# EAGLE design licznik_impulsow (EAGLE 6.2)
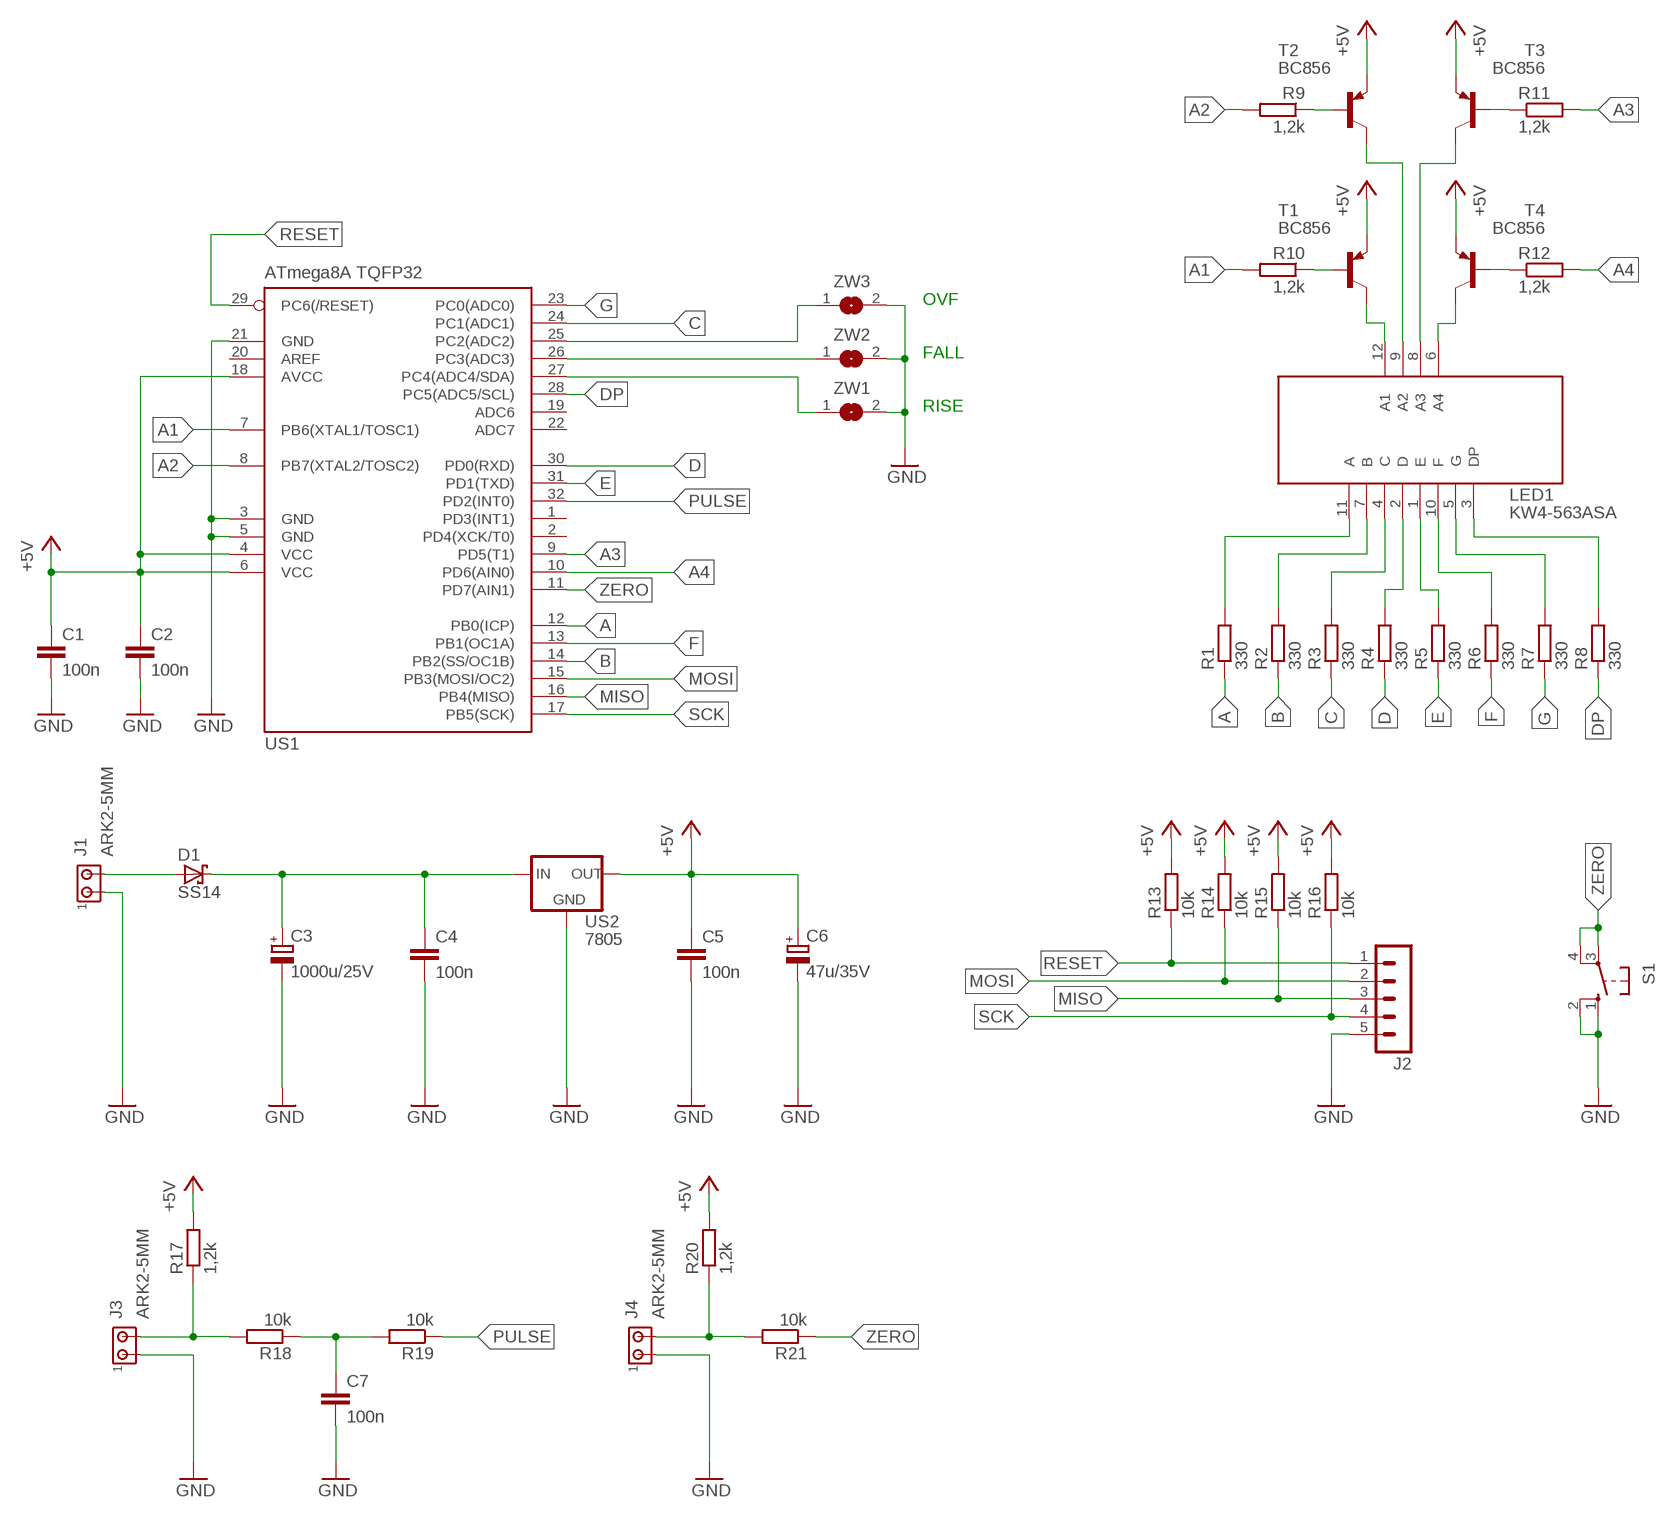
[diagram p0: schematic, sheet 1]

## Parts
C1  100n  C-EUC1206  [C1206]
C2  100n  C-EUC1206  [C1206]
C3  1000u/25V  CPOL-EUE5-10.5  [E5-10,5]
C4  100n  C-EUC1206  [C1206]
C5  100n  C-EUC1206  [C1206]
C6  47u/35V  CPOL-EUE2.5-5  [E2,5-5]
C7  100n  C-EUC1206  [C1206]
D1  SS14  SCHOTTKY-DIODESMD  [SMB]
J1  ARK2-5MM  [2PIN-5MM]
J2  MA05-1  [MA05-1]
J3  ARK2-5MM  [2PIN-5MM]
J4  ARK2-5MM  [2PIN-5MM]
LED1  KW4-563ASA  LED_DISP_KW4-563  [LED_DISP_KW4-563]
R1  330  R-EU_R1206  [R1206]
R2  330  R-EU_R1206  [R1206]
R3  330  R-EU_R1206  [R1206]
R4  330  R-EU_R1206  [R1206]
R5  330  R-EU_R1206  [R1206]
R6  330  R-EU_R1206  [R1206]
R7  330  R-EU_R1206  [R1206]
R8  330  R-EU_R1206  [R1206]
R9  1,2k  R-EU_R1206  [R1206]
R10  1,2k  R-EU_R1206  [R1206]
R11  1,2k  R-EU_R1206  [R1206]
R12  1,2k  R-EU_R1206  [R1206]
R13  10k  R-EU_R1206  [R1206]
R14  10k  R-EU_R1206  [R1206]
R15  10k  R-EU_R1206  [R1206]
R16  10k  R-EU_R1206  [R1206]
R17  1,2k  R-EU_R1206  [R1206]
R18  10k  R-EU_R1206  [R1206]
R19  10k  R-EU_R1206  [R1206]
R20  1,2k  R-EU_R1206  [R1206]
R21  10k  R-EU_R1206  [R1206]
S1  10-XX  [B3F-10XX]
T1  BC856  BC807-16LT1SMD  [SOT23-BEC]
T2  BC856  BC807-16LT1SMD  [SOT23-BEC]
T3  BC856  BC807-16LT1SMD  [SOT23-BEC]
T4  BC856  BC807-16LT1SMD  [SOT23-BEC]
US1  ATmega8A TQFP32  MEGA8-AI  [TQFP32-08]
US2  7805  78XXS  [78XXS]
ZW1  SJW  [SJW]
ZW2  SJW  [SJW]
ZW3  SJW  [SJW]

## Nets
+5V: C1.1 C2.1 C5.1 C6.+ R13.2 R14.2 R15.2 R16.2 R17.2 R20.2 T1.E T2.E T3.E T4.E US1.4(VCC) US1.6(VCC) US1.18(AVCC) US2.OUT
A: R1.1 US1.12(PB0(ICP))
A1: R10.2 US1.7(PB6(XTAL1/TOSC1))
A2: R9.2 US1.8(PB7(XTAL2/TOSC2))
A3: R11.2 US1.9(PD5(T1))
A4: R12.2 US1.10(PD6(AIN0))
B: R2.1 US1.14(PB2(SS/OC1B))
C: R3.1 US1.24(PC1(ADC1))
D: R4.1 US1.30(PD0(RXD))
DP: R8.1 US1.28(PC5(ADC5/SCL))
E: R5.1 US1.31(PD1(TXD))
F: R6.1 US1.13(PB1(OC1A))
G: R7.1 US1.23(PC0(ADC0))
GND: C1.2 C2.2 C3.- C4.2 C5.2 C6.- C7.2 J1.P$1 J2.5 J3.P$1 J4.P$1 S1.1(S) S1.2(S1) US1.3(GND) US1.5(GND) US1.21(GND) US2.GND ZW1.2 ZW2.2 ZW3.2
MISO: J2.3 R15.1 US1.16(PB4(MISO))
MOSI: J2.2 R14.1 US1.15(PB3(MOSI/OC2))
N$1: R10.1 T1.B
N$2: LED1.12(A1) T1.C
N$3: C7.1 R18.1 R19.2
N$4: US1.26(PC3(ADC3)) ZW2.1
N$5: US1.25(PC2(ADC2)) ZW3.1
N$6: US1.27(PC4(ADC4/SDA)) ZW1.1
N$7: LED1.11(A) R1.2
N$8: LED1.7(B) R2.2
N$9: LED1.4(C) R3.2
N$10: LED1.2(D) R4.2
N$11: LED1.1(E) R5.2
N$12: LED1.10(F) R6.2
N$13: LED1.5(G) R7.2
N$14: LED1.3(DP) R8.2
N$15: D1.A J1.P$2
N$16: C3.+ C4.1 D1.C US2.IN
N$17: J4.P$2 R20.1 R21.2
N$25: R9.1 T2.B
N$26: LED1.9(A2) T2.C
N$27: R11.1 T3.B
N$28: LED1.8(A3) T3.C
N$29: R12.1 T4.B
N$30: LED1.6(A4) T4.C
N$35: J3.P$2 R17.1 R18.2
PULSE: R19.1 US1.32(PD2(INT0))
RESET: J2.1 R13.1 US1.29(PC6(/RESET))
SCK: J2.4 R16.1 US1.17(PB5(SCK))
ZERO: R21.1 S1.3(P) S1.4(P1) US1.11(PD7(AIN1))
Unconnected: US1.1(PD3(INT1)) US1.2(PD4(XCK/T0)) US1.19(ADC6) US1.20(AREF) US1.22(ADC7)

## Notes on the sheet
- OVF
- FALL
- RISE

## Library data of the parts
C1 C2 C4 C5 C7 = rcl:C-EU: CAPACITOR, European symbol
C3 C6 = rcl:CPOL-EU: POLARIZED CAPACITOR, European symbol
D1 = diode:SCHOTTKY-DIODE: Schottky Diode
J1 J3 J4 = zlacza_futrzak:ARK2: ARK 2
J2 = zlacza_futrzak:MA05-1: PIN HEADER; OC_FARNELL: unknown; OC_NEWARK: unknown
LED1 = inne_futrzak:LED_DISP_KW4-563
R1-R21 = rcl:R-EU_: RESISTOR, European symbol
S1 = switch-omron:10-XX: OMRON SWITCH; MPN: B3F-1000; OC_FARNELL: 176432; OC_NEWARK: 36M3542
T1-T4 = transistor-pnp:BC807*: PNP Transistror
US1 = atmel:MEGA8: MICROCONTROLLER 8 Kbytes FLASH, 1 kbytes SRAM, 512 bytes EEPROM, USART, 6-channel 10 bit ADC, 2-channel 8 bit ADC Pin compatible with Atmega48, ATMega88, ATMega168 Source: avr.lbr; MPN: ATMEGA8-16AU; OC_FARNELL: 9171371; OC_NEWARK: 73M8863
US2 = v-reg:78XXS: VOLTAGE REGULATOR
ZW1-ZW3 = jumper:SJ: SMD solder JUMPER

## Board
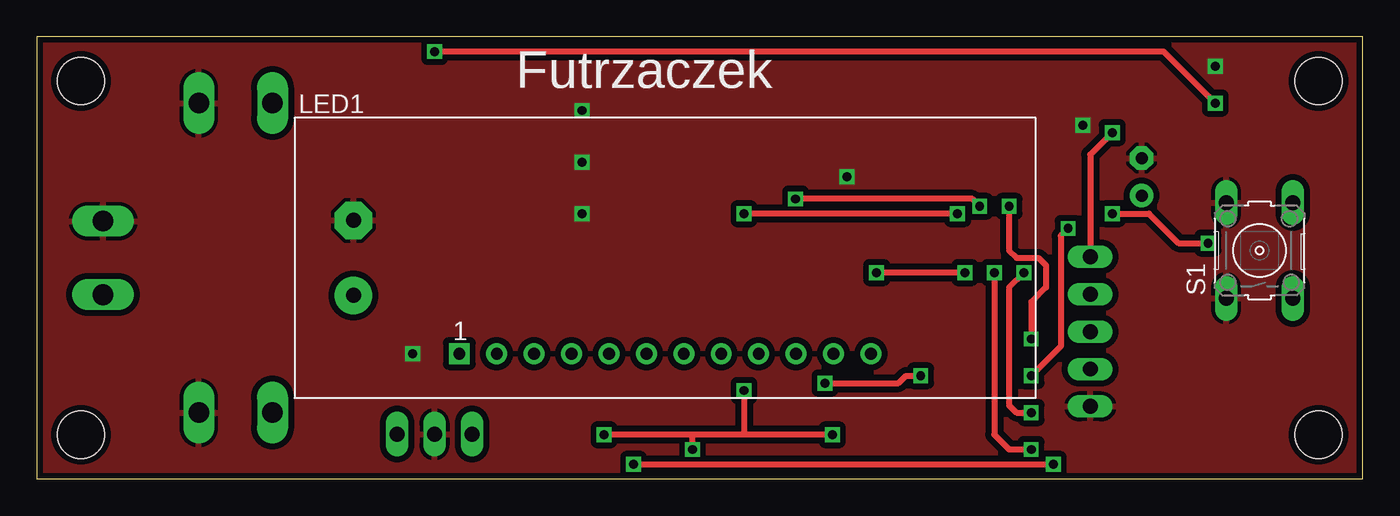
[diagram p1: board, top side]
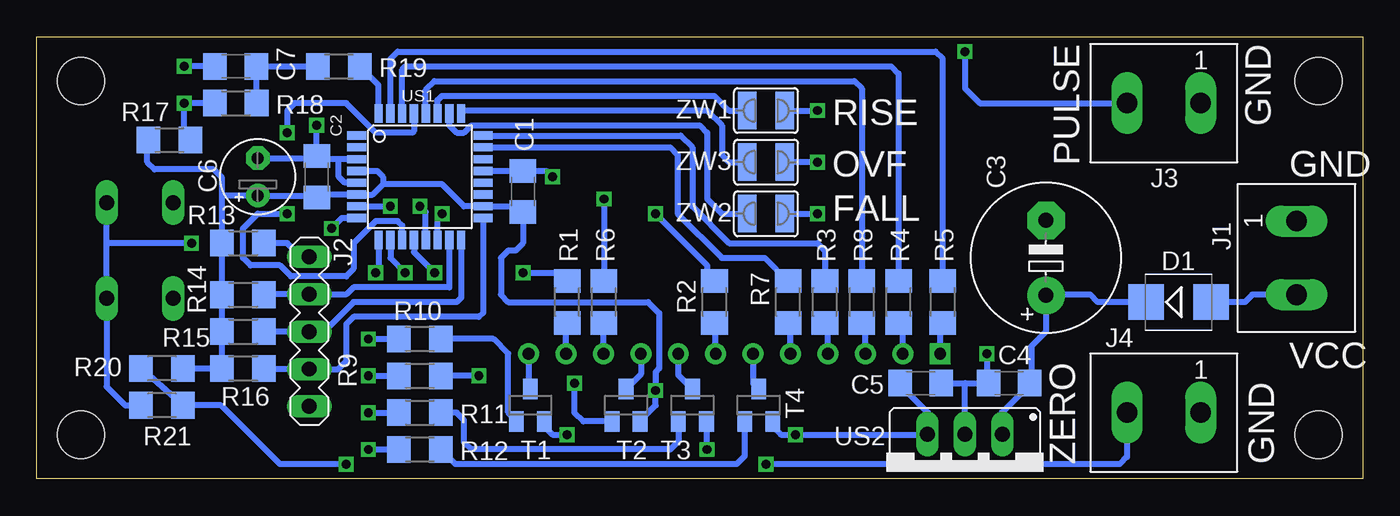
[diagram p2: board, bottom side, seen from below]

Size 90 x 30 mm. Coordinates in mm from the lower left corner, seen from the top.
Outline: 0,0 90,0 90,30 0,30 0,0
Copper layers (1*16): Top 0.035mm / dielectric 1.5mm / Bottom 0.035mm
Design rules: minimum track width 10mil, minimum drill 23mil, track to track 8mil, track to pad 8mil, pad to pad 8mil, via to via 8mil, smd to smd 8mil, copper to edge 10mil, drill to drill 8mil, minimum pad ring 10mil, minimum via ring 8mil, stop-mask expansion 4mil, vias tented up to drill 0mil, thermal gap 10mil
Holes 3.2 mm at 87,3 87,27 3,3 3,27

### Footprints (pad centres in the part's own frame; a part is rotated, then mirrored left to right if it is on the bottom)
C1206 = smd 1.6 x 1.8: 1 -1.4,0; 2 1.4,0
E5-10,5 = drill 1.016 pad 2.54: + -2.54,0 | drill 1.016 pad 2.54 octagon: - 2.54,0
E2,5-5 = drill 0.813 pad 1.6: + -1.27,0 | drill 0.813 pad 1.6 octagon: - 1.27,0
SMB = smd 2.4 x 2.4: A 2.2,0; C -2.2,0
2PIN-5MM = drill 1.4 long: P$1 -2.5,0; P$2 2.5,0
MA05-1 = drill 1.016 long: 1 -5.08,0; 2 -2.54,0; 3 0,0; 4 2.54,0; 5 5.08,0
LED_DISP_KW4-563 = drill 0.8 pad 1.422 square: 1 11.18,3 | drill 0.8 pad 1.422: 2 13.72,3; 3 16.26,3; 4 18.8,3; 5 21.34,3; 6 23.88,3; 7 26.42,3; 8 28.96,3; 9 31.5,3; 10 34.04,3; 11 36.58,3; 12 39.12,3
R1206 = smd 1.6 x 1.803: 1 -1.422,0; 2 1.422,0
B3F-10XX = drill 1.016 long: 1 -3.251,2.261; 2 3.251,2.261; 3 -3.251,-2.261; 4 3.251,-2.261
SOT23-BEC = smd 1 x 1.4: B -0.95,-1.1; C 0,1.1; E 0.95,-1.1
TQFP32-08 = smd 1.27 x 0.559: 1 -4.293,2.8; 2 -4.293,2; 3 -4.293,1.2; 4 -4.293,0.4; 5 -4.293,-0.4; 6 -4.293,-1.2; 7 -4.293,-2; 8 -4.293,-2.8; 17 4.293,-2.8; 18 4.293,-2; 19 4.293,-1.2; 20 4.293,-0.4; 21 4.293,0.4; 22 4.293,1.2; 23 4.293,2; 24 4.293,2.8 | smd 0.559 x 1.27: 9 -2.8,-4.293; 10 -2,-4.293; 11 -1.2,-4.293; 12 -0.4,-4.293; 13 0.4,-4.293; 14 1.2,-4.293; 15 2,-4.293; 16 2.8,-4.293; 25 2.8,4.293; 26 2,4.293; 27 1.2,4.293; 28 0.4,4.293; 29 -0.4,4.293; 30 -1.2,4.293; 31 -2,4.293; 32 -2.8,4.293
78XXS = drill 1.016 long: GND 0,-2.54; IN -2.54,-2.54; OUT 2.54,-2.54
SJW = smd 1.27 x 2.54: 1 -1.27,0; 2 1.27,0

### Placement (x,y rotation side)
C1  57,19.5 90 bottom
C2  71,20.5 90 bottom
C3  21.5,15 90 bottom
C4  24,6.5 180 bottom
C5  30,6.5 0 bottom
C6  75,20.5 90 bottom
C7  76.5,28 180 bottom
D1  12.5,12 0 bottom
J1  4.5,15 270 bottom
J2  71.5,10 270 bottom
J3  13.5,25.5 180 bottom
J4  13.5,4.5 180 bottom
LED1  17.5,5.5 0 top
R1  54,12 270 bottom
R2  44,12 270 bottom
R3  36.5,12 270 bottom
R4  31.5,12 270 bottom
R5  28.5,12 270 bottom
R6  51.5,12 270 bottom
R7  39,12 270 bottom
R8  34,12 270 bottom
R9  64,7 180 bottom
R10  64,9.5 180 bottom
R11  64,4.5 180 bottom
R12  64,2 180 bottom
R13  76,16 180 bottom
R14  76,12.5 180 bottom
R15  76,10 180 bottom
R16  76,7.5 180 bottom
R17  81,23 180 bottom
R18  76.5,25.5 180 bottom
R19  69.5,28 180 bottom
R20  81.5,7.5 0 bottom
R21  81.5,5 0 bottom
S1  83,15.5 90 top
T1  56.5,5 0 bottom
T2  50,5 0 bottom
T3  45.5,5 0 bottom
T4  41,5 0 bottom
US1  64,20.5 0 bottom
US2  27,0.5 180 bottom
ZW1  40.5,25 0 bottom
ZW2  40.5,18 0 bottom
ZW3  40.5,21.5 0 bottom

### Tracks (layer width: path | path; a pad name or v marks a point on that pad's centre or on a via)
+5V  (via drill 0.6)
  Top 0.406: v54,3 48,3 | 48,3 44.5,3 | 44.5,3 v38.5,3 | v44.5,2 44.5,3 | v48,6 48,3
  Bottom 0.406: 66.5,20 67.2,19.3 US1.6 70.8,19.3 C2.1 71.13,19.23 C6.+ 77.42,19.23 | US1.4 66.9,20.9 66.5,20.5 66.5,20 | 66.5,20 62.5,20 61,18.5 US1.18 57.4,18.5 C1.1 57,16 57.5,15.5 58,15.5 58.5,15 58.5,12.5 58,12 48.5,12 47.75,11.25 47.75,7.5 48,7.25 v48,6 48,5 49.05,3.95 T2.E | 77.42,19.23 R13.2 R14.2 R15.2 R16.2 R20.2 | T1.E 55.55,3.55 55,3 v54,3 | T4.E 40.05,3.55 39.5,3 v38.5,3 29.58,3 US2.OUT 29.5,3.08 29.5,4.5 31.4,6.4 C5.1 | T3.E 44.55,2.05 v44.5,2 | R17.2 82.5,22.92 82.5,21.5 82,21 78,21 77.42,20.42 77.42,19.23
A  (via drill 0.6)
  Top 0.406: v63,14 v57,14
  Bottom 0.406: US1.12 64.4,15.4 v63,14 | v57,14 54.58,14 R1.1
A1  (via drill 0.6)
  Top 0.406: v66,18.5 66,15.5 66.5,15 68,15 68.5,14.5 68.5,13 67.5,12 v67.5,9.5
  Bottom 0.406: US1.7 v66,18.5 | v67.5,9.5 R10.2
A2  (via drill 0.6)
  Top 0.406: v70,17 69.5,16.5 69.5,9 v67.5,7
  Bottom 0.406: US1.8 69.3,17.7 v70,17 | v67.5,7 R9.2
A3  (via drill 0.6)
  Top 0.406: v67,14 66,13 66,5 66.5,4.5 v67.5,4.5
  Bottom 0.406: US1.9 66.8,14.2 v67,14 | v67.5,4.5 R11.2
A4  (via drill 0.6)
  Top 0.406: v65,14 65,3 66,2 v67.5,2
  Bottom 0.406: US1.10 66,15 v65,14 | v67.5,2 R12.2
B  (via drill 0.6)
  Top 0.406: v62.5,18 v48,18
  Bottom 0.406: US1.14 62.8,17.7 v62.5,18 | v48,18 44.5,14.5 44.5,13.92 R2.1
C
  Bottom 0.406: US1.24 46.3,23.3 45.5,22.5 45.5,18.5 43,16 37,16 36.5,15.5 R3.1
D
  Bottom 0.406: US1.30 65.2,27.8 65,28 32,28 31.5,27.5 R4.1
DP
  Bottom 0.406: US1.28 63.6,26.4 63,27 34.5,27 34,26.5 R8.1
E
  Bottom 0.406: US1.31 66,28.5 65.5,29 29,29 28.5,28.5 R5.1
F  (via drill 0.6)
  Top 0.406: v64,18.5 63.5,19 v51.5,19
  Bottom 0.406: US1.13 63.6,18.1 v64,18.5 | v51.5,19 R6.1
G
  Bottom 0.406: US1.23 47,22.5 46.5,22 46.5,18 43.5,15 40.58,15 R7.1
GND  (via drill 0.6)
  Bottom 0.406: ZW1.2 v37,25 | v37,21.5 ZW3.2 | ZW2.2 v37,18 | US1.21 C1.2 55.4,20.9 v55,20.5 | 69.5,21.7 US1.3 70.7,21.7 71,22 v71,24 | 69.5,21.7 70.8,21.7 C2.2 71.13,21.77 C6.- | US1.5 69.1,20.1 69.5,20.5 69.5,21.7 | US2.GND 27,6.5 | 27,6.5 C4.2 25.5,6.6 v25.5,8.5 | C5.2 27,6.5 | C7.2 v80,28
  pour Top (isolate 0.406): 0,0 90,0 90,30 0,30
MISO
  Bottom 0.406: US1.16 61.2,12.3 61.5,12 68.5,12 70.5,10 J2.3 R15.1
MOSI
  Bottom 0.406: US1.15 62,13 68.5,13 68.96,12.54 J2.2 74.54,12.54 R14.1
N$1
  Bottom 0.406: T1.B 57.45,3.95 58,4.5 58,8.5 59,9.5 R10.1
N$2
  Bottom 0.406: LED1.12 56.62,6.22 T1.C
N$3
  Bottom 0.406: R18.1 75.08,27.98 C7.1 R19.2
N$4
  Bottom 0.406: US1.26 62,24 61.5,23.5 61,23.5 60.5,24 45,24 44.5,23.5 44.5,19 43.5,18 ZW2.1
N$5
  Bottom 0.406: ZW3.1 43,21.5 43.5,22 43.5,24 44.5,25 60.99,25 US1.25
N$6
  Bottom 0.406: US1.27 62.8,25.7 62.5,26 44,26 43,25 ZW1.1
N$7
  Bottom 0.406: LED1.11 54.08,11 R1.2
N$8
  Bottom 0.406: LED1.7 43.92,11 R2.2
N$9
  Bottom 0.406: LED1.4 36.3,10.88 R3.2
N$10
  Bottom 0.406: LED1.2 31.22,10.8 R4.2
N$11
  Bottom 0.406: LED1.1 28.68,10.9 R5.2
N$12
  Bottom 0.406: LED1.10 51.54,11.04 R6.2
N$13
  Bottom 0.406: LED1.5 38.84,10.92 R7.2
N$14
  Bottom 0.406: LED1.3 33.76,10.84 R8.2
N$15
  Bottom 0.406: J1.P$2 7.5,12.5 8,12 D1.A
N$16
  Bottom 0.406: US2.IN 24.5,3.08 24.5,4.5 22.6,6.4 C4.1 22.5,6.6 22.5,9 21.5,10 C3.+ 21.46,12.5 18.5,12.5 18,12 D1.C
N$17  (via drill 0.6)
  Top 0.406: v40.5,1 v69,1
  Bottom 0.406: R20.1 R21.2 77.5,5 73.5,1 v69,1 | J4.P$2 16,1.5 16.5,1 v40.5,1
N$25  (via drill 0.6)
  Top 0.406: v53.5,6.5 58.5,6.5 59,7 v60,7
  Bottom 0.406: T2.B 52.9,3.9 53.5,4.5 v53.5,6.5 | v60,7 R9.1
N$26
  Bottom 0.406: LED1.9 49,7.1 T2.C
N$27
  Bottom 0.406: T3.B 46.45,2.55 47,2 60.5,2 61,2.5 61,4 61.5,4.5 R11.1
N$28
  Bottom 0.406: LED1.8 46.46,7.06 T3.C
N$29
  Bottom 0.406: T4.B 41.95,1.55 42.5,1 61.58,1 R12.1
N$30
  Bottom 0.406: LED1.6 41.38,6.48 T4.C
N$35  (via drill 0.6)
  Top 0.406: v80,25.5 76.5,29 v27,29
  Bottom 0.406: R17.1 79.58,23.08 80,23.5 v80,25.5 R18.2 | v27,29 27,26.5 26,25.5 J3.P$2
PULSE
  Bottom 0.406: US1.32 66.8,26.72 R19.1
RESET  (via drill 0.6)
  Top 0.406: v73,23.5 71.5,22 J2.1
  Bottom 0.406: J2.1 72.08,15.08 73,16 R13.1 | US1.29 64.4,23.6 64.5,23.5 67,23.5 69,25.5 72.5,25.5 73,25 v73,23.5
SCK
  Bottom 0.406: US1.17 59.71,11.29 60,11 68.5,11 69,10.5 69,8 69.54,7.46 J2.4 74.54,7.46 R16.1
ZERO  (via drill 0.6)
  Top 0.406: v73,18 75.5,18 77.5,16 v79.5,16
  Bottom 0.406: US1.11 65.2,17.2 65.5,17.5 67,17.5 68.5,16 68.5,14.25 69,13.75 72.75,13.75 73.5,14.5 75.5,14.5 76,15 76,17 75,18 v73,18 | v79.5,16 85.26,16 | 85.26,16 S1.3 85.26,6.26 84,5 R21.1 | 85.26,16 S1.4

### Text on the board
tPlace: Futrzaczek
bPlace: GND | PULSE | RISE | GND | OVF | FALL | VCC | GND | ZERO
